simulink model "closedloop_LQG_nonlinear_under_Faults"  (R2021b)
settings: Solver=ode45  StartTime=0.0  StopTime=1500  RelTol=1e-10  AbsTol=1e-10
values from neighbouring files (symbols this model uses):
  Atap = [-atap/A1*sqrt(2*g)    0   0   0    [initial_quadtank_nonlinear.m]
  Dcup = diag([1/A1 1/A2 1/A3 1/A4])    [initial_quadtank_nonlinear.m]
  flag_DoS_attack = 0    [set_attacks.m]
  flag_replay_attack = 0    [set_attacks.m]
  flag_sensor_attack = 0    [set_attacks.m]
  mag_DoS_attack = 0.96    [set_attacks.m]
  Qn = eye(size(G,2))*0.01    [initialize_closed_loop_system.m]    (also in Load_Data.m; run_experiment.m = eye(size(G,2))*0)
  Rn = eye(p)*0.0025    [initialize_closed_loop_system.m]    (also in Load_Data.m; run_experiment.m = eye(p)*0)
  sys_tmp = ss(A*1,[B G]*1,C,[D H],Ts)    [initialize_closed_loop_system.m]    (also in Load_Data.m = ss(A,[B Ba],[C; Cp],[D Da; Dp, Dp, zeros(size(Dp,1),ny)],Ts))
  T_attack_start = 100    [set_attacks.m]
  Ts = 2    [initialize_closed_loop_system.m]    (also in Load_Data.m = 0; run_experiment.m = sysmp_d.Ts)
  u0 = [u10;u20]    [initial_quadtank_nonlinear.m]    (also in setup_quadtank_nonlinear.m)
  ub = 25    [msfcn_quadtank_nonlinear.m]    (also in initialize_closed_loop_system.m = 15; Load_Data.m = 15)
  ul = 0    [initialize_closed_loop_system.m]    (also in Load_Data.m)
  x0 = x.^2    [initial_quadtank_nonlinear.m]    (also in setup_quadtank_nonlinear.m)
  y0 = kc*x0(1:2)    [initial_quadtank_nonlinear.m]    (also in setup_quadtank_nonlinear.m)
undefined symbols (not defined in the file or in its folder): An, Bn, Klq
libraries: simulink x3, cstblocks x2

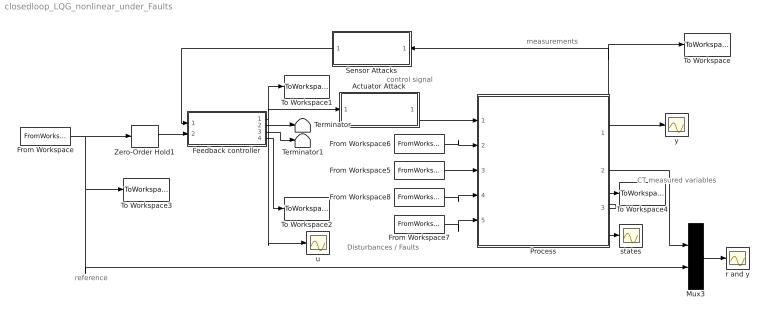
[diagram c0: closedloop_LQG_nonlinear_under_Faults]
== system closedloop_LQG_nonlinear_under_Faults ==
  note: control signal
  note: CT measured variables
  note: reference
  note: measurements
  note: Disturbances / Faults
  Actuator Attack : Subsystem
  Feedback controller : Subsystem  TreatAsAtomicUnit=on
  From Workspace : FromWorkspace  VariableName=ref  Interpolate=off  OutputAfterFinalValue=Holding final value
  From Workspace5 : FromWorkspace  VariableName=dtap  Interpolate=off  OutputAfterFinalValue=Holding final value
  From Workspace6 : FromWorkspace  VariableName=dcup  Interpolate=off  OutputAfterFinalValue=Holding final value
  From Workspace7 : FromWorkspace  VariableName=fsensor  Interpolate=off  OutputAfterFinalValue=Holding final value
  From Workspace8 : FromWorkspace  VariableName=factuator  Interpolate=off  OutputAfterFinalValue=Holding final value
  Mux3 : Mux  Inputs=2
  Process : Subsystem
  Sensor Attacks : Subsystem
  Terminator : Terminator
  Terminator1 : Terminator
  To Workspace : ToWorkspace  VariableName=measurement  SaveFormat=Timeseries  SampleTime=Ts
  To Workspace1 : ToWorkspace  VariableName=control_signal  SaveFormat=Timeseries  SampleTime=Ts
  To Workspace2 : ToWorkspace  VariableName=residuals  SaveFormat=Timeseries  SampleTime=Ts
  To Workspace3 : ToWorkspace  VariableName=reference  SaveFormat=Timeseries  SampleTime=Ts
  To Workspace4 : ToWorkspace  VariableName=state_signals  SaveFormat=Timeseries  SampleTime=Ts
  Zero-Order Hold1 : ZeroOrderHold  SampleTime=Ts
  r and y : Scope
  states : Scope
  u : Scope
  y : Scope
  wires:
  From Workspace/1 -> Mux3/2, To Workspace3/1, Zero-Order Hold1/1
  Zero-Order Hold1/1 -> Feedback controller/2(ref)
  Mux3/1 -> r and y/1
  Process/1(y_meas) -> To Workspace/1, Sensor Attacks/1(In1), y/1
  From Workspace6/1 -> Process/2(pulse disturbance)
  From Workspace5/1 -> Process/3(leakage fault)
  From Workspace8/1 -> Process/4(actuator fault)
  From Workspace7/1 -> Process/5(sensor fault)
  Process/2(y_continuous) -> Mux3/1
  Feedback controller/4(residuals) -> To Workspace2/1
  Process/3(x internal) -> states/1, To Workspace4/1
  Sensor Attacks/1(Out1) -> Feedback controller/1(y)
  Actuator Attack/1(Out1) -> Process/1(u2)
  Feedback controller/1(u) -> Actuator Attack/1(In1), To Workspace1/1, u/1
  Feedback controller/2(D y) -> Terminator/1
  Feedback controller/3(D y_est) -> Terminator1/1

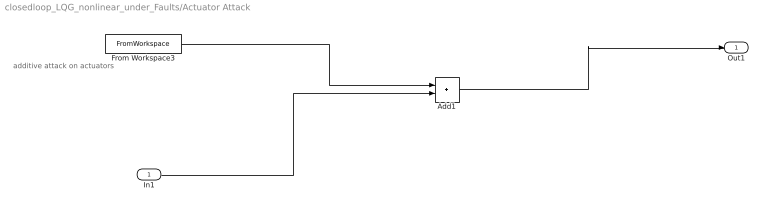
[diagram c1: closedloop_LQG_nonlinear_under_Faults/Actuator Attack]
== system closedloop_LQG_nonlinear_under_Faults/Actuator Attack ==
  note: additive attack on actuators
  In1 : Inport
  Add1 : Sum
  From Workspace3 : FromWorkspace  VariableName=undetectable_attack  SampleTime=Ts  Interpolate=off  OutputAfterFinalValue=Holding final value
  Out1 : Outport  VectorParamsAs1DForOutWhenUnconnected=off
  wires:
  Add1/1 -> Out1/1
  In1/1 -> Add1/2
  From Workspace3/1 -> Add1/1

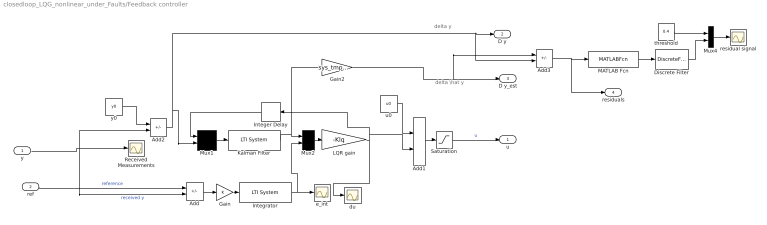
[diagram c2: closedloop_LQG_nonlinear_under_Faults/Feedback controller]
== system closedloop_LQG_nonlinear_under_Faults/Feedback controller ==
  note: delta \hat y
  note: delta y
  y : Inport
  ref : Inport  Port=2
  Add : Sum  Inputs=+-
  Add1 : Sum
  Add2 : Sum  Inputs=-+
  Add3 : Sum  Inputs=-+
  Discrete Filter : DiscreteFilter  Numerator=[0 (1-0.05)]  Denominator=[1 -0.05]  SampleTime=Ts
  Gain : Gain
  Gain2 : Gain  Gain=sys_tmp.c  Multiplication=Matrix(K*u) (u vector)
  Integer Delay : Delay  DelayLength=1
  Integrator : cstblocks/LTI System  sys=sys_int  IC=0
  Kalman Filter : cstblocks/LTI System  sys=F  IC=0
  LQR gain : Gain  Gain=-Klq  Multiplication=Matrix(K*u) (u vector)
  MATLAB Fcn : MATLABFcn  MATLABFcn=norm(u,2)
  Mux1 : Mux  Inputs=2
  Mux2 : Mux  Inputs=2
  Mux4 : Mux  Inputs=2
  Received Measurements : Scope
  Saturation : Saturate  UpperLimit=ub  LowerLimit=ul
  du : Scope
  e_int : Scope
  residual signal : Scope
  threshold : Constant  Value=0.4  VectorParams1D=off
  u0 : Constant  Value=u0  VectorParams1D=off
  y0 : Constant  Value=y0  VectorParams1D=off  SampleTime=Ts
  u : Outport  VectorParamsAs1DForOutWhenUnconnected=off
  D y : Outport  Port=2  VectorParamsAs1DForOutWhenUnconnected=off
  D y_est : Outport  Port=3  VectorParamsAs1DForOutWhenUnconnected=off
  residuals : Outport  Port=4  VectorParamsAs1DForOutWhenUnconnected=off
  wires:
  Add2/1 -> Add3/2, D y/1, Mux1/2
  y0/1 -> Add2/1
  Mux2/1 -> LQR gain/1
  Integrator/1 -> Mux2/2, e_int/1
  Mux1/1 -> Kalman Filter/1
  Add1/1 -> Saturation/1
  Add/1 -> Gain/1
  u0/1 -> Add1/1
  ref/1 -> Add/1  "reference"
  LQR gain/1 -> Add1/2, Integer Delay/1, du/1
  Gain/1 -> Integrator/1
  y/1 -> Add/2, Add2/2, Received Measurements/1  "received y"
  Integer Delay/1 -> Mux1/1
  Kalman Filter/1 -> Gain2/1, Mux2/1
  Gain2/1 -> Add3/1, D y_est/1
  Saturation/1 -> u/1  "u"
  Add3/1 -> residuals/1, MATLAB Fcn/1
  Mux4/1 -> residual signal/1
  threshold/1 -> Mux4/1
  MATLAB Fcn/1 -> Discrete Filter/1
  Discrete Filter/1 -> Mux4/2

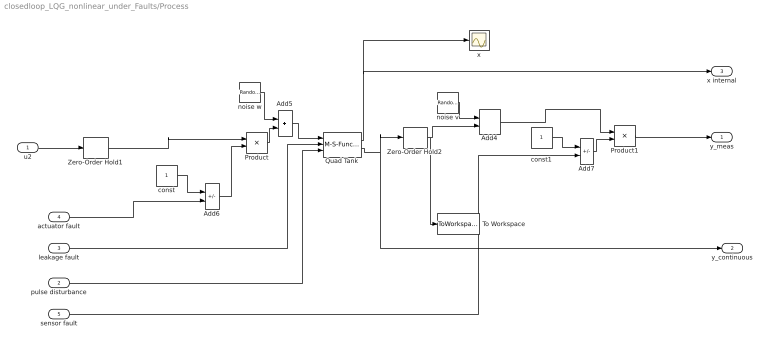
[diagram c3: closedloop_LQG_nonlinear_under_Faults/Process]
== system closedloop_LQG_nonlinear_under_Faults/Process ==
  u2 : Inport
  pulse disturbance : Inport  Port=2
  leakage fault : Inport  Port=3
  actuator fault : Inport  Port=4
  sensor fault : Inport  Port=5
  Add4 : Sum
  Add5 : Sum
  Add6 : Sum  Inputs=+-
  Add7 : Sum  Inputs=+-
  Product : Product
  Product1 : Product
  Quad Tank : M-S-Function  FunctionName=msfcn_quadtank_nonlinear  Parameters=x0,An,Bn,Atap,Dcup
  To Workspace : ToWorkspace  VariableName=measurement_no_noise  SaveFormat=Timeseries  SampleTime=Ts
  Zero-Order Hold1 : ZeroOrderHold  SampleTime=Ts
  Zero-Order Hold2 : ZeroOrderHold  SampleTime=Ts
  const : Constant  VectorParams1D=off
  const1 : Constant  VectorParams1D=off  SampleTime=Ts
  noise v : RandomNumber  Mean=0*diag(Rn)  Variance=diag(Rn)*1  Seed=[0;10]  SampleTime=Ts  VectorParams1D=off
  noise w : RandomNumber  Mean=0*diag(Qn)  Variance=diag(Qn)*1  Seed=[0;20]  SampleTime=Ts  VectorParams1D=off
  x : Scope
  y_meas : Outport  VectorParamsAs1DForOutWhenUnconnected=off
  y_continuous : Outport  Port=2  VectorParamsAs1DForOutWhenUnconnected=off
  x internal : Outport  Port=3  VectorParamsAs1DForOutWhenUnconnected=off
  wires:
  noise w/1 -> Add5/1
  Zero-Order Hold2/1 -> To Workspace/1, Add4/2
  Quad Tank/2 -> y_continuous/1, Zero-Order Hold2/1
  Add5/1 -> Quad Tank/1
  const1/1 -> Add7/1
  const/1 -> Add6/1
  Product1/1 -> y_meas/1
  Add7/1 -> Product1/2
  Add4/1 -> Product1/1
  noise v/1 -> Add4/1
  leakage fault/1 -> Quad Tank/2
  sensor fault/1 -> Add7/2
  Product/1 -> Add5/2
  Add6/1 -> Product/2
  Quad Tank/1 -> x internal/1, x/1
  actuator fault/1 -> Add6/2
  pulse disturbance/1 -> Quad Tank/3
  u2/1 -> Zero-Order Hold1/1
  Zero-Order Hold1/1 -> Product/1

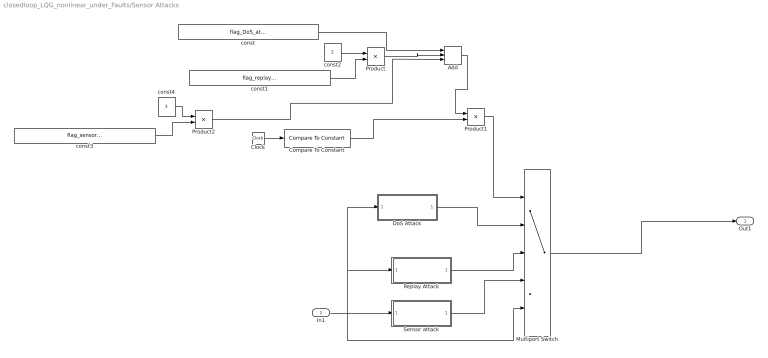
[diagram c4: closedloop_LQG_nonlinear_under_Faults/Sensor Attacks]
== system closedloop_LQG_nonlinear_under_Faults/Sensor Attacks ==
  In1 : Inport
  Add : Sum  Inputs=+++
  Clock : Clock
  Compare To Constant : simulink/Logic and Bit Operations/Compare To Constant  relop=>=  const=T_attack_start  OutDataTypeStr=boolean
  DoS Attack : Subsystem
  Multiport Switch : MultiPortSwitch  DataPortForDefault=Additional data port  DiagnosticForDefault=None
  Product : Product
  Product1 : Product
  Product2 : Product
  Replay Attack : Subsystem
  Sensor attack : Subsystem
  const : Constant  Value=flag_DoS_attack  VectorParams1D=off
  const1 : Constant  Value=flag_replay_attack  VectorParams1D=off
  const2 : Constant  Value=2  VectorParams1D=off
  const3 : Constant  Value=flag_sensor_attack  VectorParams1D=off
  const4 : Constant  Value=3  VectorParams1D=off
  Out1 : Outport  VectorParamsAs1DForOutWhenUnconnected=off
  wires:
  Multiport Switch/1 -> Out1/1
  In1/1 -> Sensor attack/1(In1), Multiport Switch/5, Replay Attack/1(In1), DoS Attack/1(In1)
  DoS Attack/1(Out1) -> Multiport Switch/2
  Replay Attack/1(Out1) -> Multiport Switch/3
  const2/1 -> Product/1
  const1/1 -> Product/2
  const/1 -> Add/1
  Product/1 -> Add/2
  Add/1 -> Product1/1
  Product1/1 -> Multiport Switch/1
  Clock/1 -> Compare To Constant/1
  Compare To Constant/1 -> Product1/2
  Sensor attack/1(Out1) -> Multiport Switch/4
  const4/1 -> Product2/1
  const3/1 -> Product2/2
  Product2/1 -> Add/3

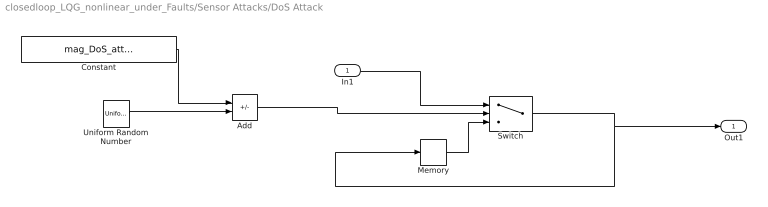
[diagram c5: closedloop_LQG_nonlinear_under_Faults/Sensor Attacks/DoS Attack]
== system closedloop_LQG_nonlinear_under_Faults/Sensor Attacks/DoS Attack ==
  In1 : Inport
  Add : Sum  Inputs=-+
  Constant : Constant  Value=mag_DoS_attack
  Memory : Memory
  Switch : Switch
  Uniform Random Number : UniformRandomNumber  Minimum=0  SampleTime=Ts
  Out1 : Outport  VectorParamsAs1DForOutWhenUnconnected=off
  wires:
  Add/1 -> Switch/2
  Memory/1 -> Switch/3
  In1/1 -> Switch/1
  Switch/1 -> Memory/1, Out1/1
  Constant/1 -> Add/1
  Uniform Random Number/1 -> Add/2

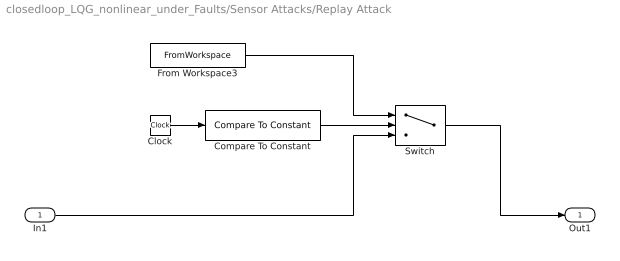
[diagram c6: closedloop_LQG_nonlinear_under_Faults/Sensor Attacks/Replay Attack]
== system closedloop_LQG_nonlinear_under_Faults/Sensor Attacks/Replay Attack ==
  In1 : Inport
  Clock : Clock
  Compare To Constant : simulink/Logic and Bit Operations/Compare To Constant  relop=>=  const=T_attack_start  OutDataTypeStr=boolean
  From Workspace3 : FromWorkspace  VariableName=recorded_measurements  SampleTime=Ts  Interpolate=off  OutputAfterFinalValue=Holding final value
  Switch : Switch  Criteria=u2 > Threshold
  Out1 : Outport  VectorParamsAs1DForOutWhenUnconnected=off
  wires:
  Clock/1 -> Compare To Constant/1
  Compare To Constant/1 -> Switch/2
  Switch/1 -> Out1/1
  In1/1 -> Switch/3
  From Workspace3/1 -> Switch/1

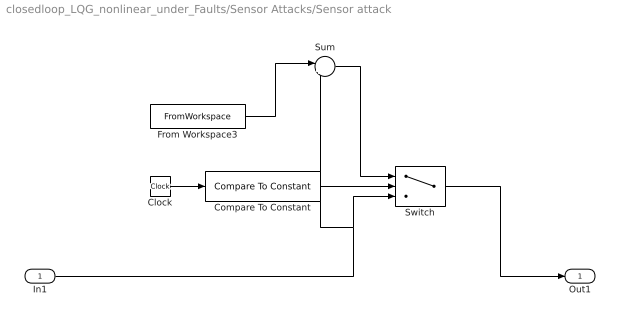
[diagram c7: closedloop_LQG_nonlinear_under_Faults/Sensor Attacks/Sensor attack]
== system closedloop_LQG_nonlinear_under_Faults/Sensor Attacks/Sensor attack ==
  In1 : Inport
  Clock : Clock
  Compare To Constant : simulink/Logic and Bit Operations/Compare To Constant  relop=>=  const=T_attack_start  OutDataTypeStr=boolean
  From Workspace3 : FromWorkspace  VariableName=undetectable_sensor_attack  SampleTime=Ts  Interpolate=off  OutputAfterFinalValue=Holding final value
  Sum : Sum  Inputs=|++
  Switch : Switch  Criteria=u2 > Threshold
  Out1 : Outport  VectorParamsAs1DForOutWhenUnconnected=off
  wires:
  Clock/1 -> Compare To Constant/1
  Compare To Constant/1 -> Switch/2
  Switch/1 -> Out1/1
  In1/1 -> Sum/2, Switch/3
  From Workspace3/1 -> Sum/1
  Sum/1 -> Switch/1
